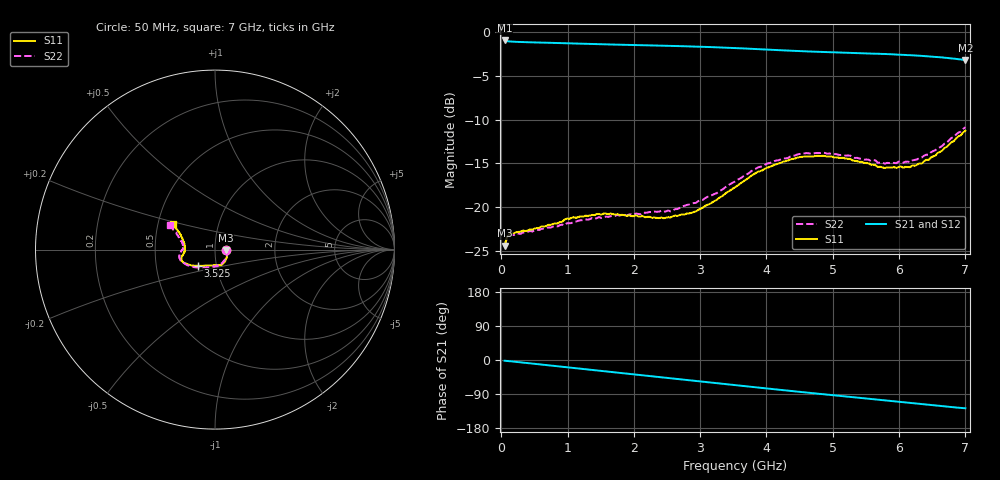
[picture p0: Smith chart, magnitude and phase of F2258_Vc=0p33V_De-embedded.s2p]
! Integrated Device Technology
! Corporate Headquarters
! 6024 Silver Creek Valley Road
! San Jose, CA 95138  USA
! Phone:  1-408-284-8200
! Toll Free:  1-800-223-1366
! Webpage:  http://www.idt.com/
! Timing and RF Division
! 515 Groton Road, Suite 102
! Westford, MA 01886-6024
! Device:  F2258
! Description: Voltage Variable RF Attenuator
! Frequency:  50.0 -  6000.00 MHz
! Package:  3x3 mm Thin QFN Plastic Package: 16 pin
! Ports:  2 RF, 2 DC
!  Pin  1  = NC
!  Pin  2  = NC
!  Pin  3  = RF2  = Port 2
!  Pin  4  = GND
!  Pin  5  = Vdd
!  Pin  6  = NC
!  Pin  7  = VCTRL
!  Pin  8  = NC
!  Pin  9  = GND
!  Pin 10  = RF1  = Port 1
!  Pin 11  = NC
!  Pin 12  = NC
!  Pin 13  = NC
!  Pin 14  = NC
!  Pin 15  = NC
!  Pin 16  = NC
! Vcntrl:  0.330 Volts
! Vdd:  +3.300 Volts
! Current:  1.089 mA
! Data:  The device was measured on a the F2258 evaluation board which has
!  individual transmission lines to the RF pins.  Data was collected
!  using a calibrated network analyzer.  The evaluation board was
!  de-embedded using a TRL calibration technique.
!  The reference plane is the edge of the package pin.
! Misc:  SN 10
!  Action Tracker AT0285
! Date Measured:  2014-12-10
! Date:  2016-01-13  MJV
! Note:
!  Integrated Device Technology supplies this data as a sample of measured
!  data at the package pin for this product.  Your particular data for this
!  product may vary.
!  Data was taken at 25 degrees C.
!  Integrated Device Technology reserves the right to change this data at anytime.
!Freq_(GHz)  S11M_(dB)  S11P_(deg)  S21M_(dB)  S21P_(deg)  S12M_(dB)  S12P_(deg)  S22M_(dB)  S22P_(deg)
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# GHz S dB R 50
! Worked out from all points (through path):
!   201 points, 50 MHz to 7 GHz, reference 50 ohm
!   highest |S21| = -0.99 dB at 50 MHz (marker M1); lowest = -3.2 dB at 7 GHz (marker M2)
!   group delay of S21, straight-line fit = 50.5 ps
!   lowest |S11| = -24.4 dB at 50 MHz (marker M3), VSWR 1.13, Z = 56.4 - j0.399 ohm
!   |S11| at or under -10 dB: start of sweep to end of sweep
!   |S22| runs from -24.4 to -10.9 dB; largest |S21 - S12| = 0.00036
!   S11 on the Smith chart (normalised r, x): 50 MHz: 1.13, -0.01; 3.525 GHz: 0.82, -0.15; 7 GHz: 0.60, +0.18
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0.05  -24.37 -3.3  -0.99 -1.9  -0.99 -1.9  -24.43 -3.0
0.08475  -23.42 -5.7  -1.07 -2.5  -1.07 -2.5  -23.51 -5.3
0.15425  -22.95 -8.9  -1.12 -3.6  -1.12 -3.6  -23.14 -9.2
0.71025  -22.00 -35.8  -1.25 -14.1  -1.25 -14.1  -22.29 -37.8
0.98825  -21.29 -49.4  -1.31 -19.3  -1.31 -19.3  -21.83 -53.6
1.2315  -21.07 -57.5  -1.36 -23.8  -1.36 -23.8  -21.48 -62.6
1.6485  -20.71 -69.1  -1.45 -31.4  -1.45 -31.4  -21.01 -75.6
2.37825  -21.24 -90.1  -1.58 -44.8  -1.57 -44.8  -20.50 -93.5
2.552  -21.16 -96.0  -1.61 -48.0  -1.61 -48.0  -20.47 -98.8
2.93425  -20.47 -112.7  -1.69 -55.1  -1.69 -55.1  -19.51 -112.2
3.247  -19.17 -125.5  -1.77 -61.0  -1.77 -61.0  -18.40 -124.4
3.525  -17.73 -136.1  -1.85 -66.2  -1.85 -66.2  -17.06 -135.0
4.0115  -15.48 -150.1  -2.03 -75.2  -2.04 -75.2  -15.02 -150.5
4.46325  -14.34 -158.7  -2.19 -83.4  -2.20 -83.4  -13.98 -161.7
4.7065  -14.20 -161.9  -2.26 -87.7  -2.27 -87.7  -13.88 -165.9
5.2625  -14.48 -168.8  -2.42 -97.4  -2.42 -97.4  -14.12 -174.0
5.6795  -15.41 -175.5  -2.50 -104.6  -2.50 -104.6  -14.92 -179.5
5.85325  -15.48 -179.7  -2.56 -107.8  -2.56 -107.8  -14.95 175.9
6.166  -15.43 172.4  -2.66 -113.4  -2.67 -113.4  -14.87 169.9
6.33975  -15.02 166.0  -2.75 -116.5  -2.75 -116.5  -14.34 165.6
6.722  -13.10 154.1  -2.98 -123.1  -2.98 -123.1  -12.64 156.5
7  -11.28 148.6  -3.23 -127.4  -3.23 -127.4  -10.87 151.5
